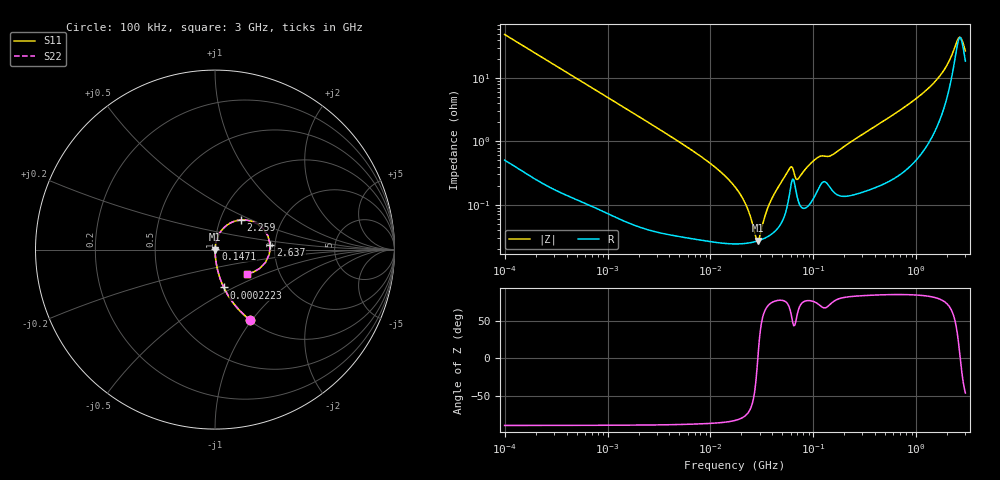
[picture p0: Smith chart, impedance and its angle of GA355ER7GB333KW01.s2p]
!Murata Part Number: GA355ER7GB333KW01
!These Parameters are Measured in Series Mode Connection
!Data Generated on Jun 19, 2026
!  o--ll--o
!Port1  Port2
!  o------o
!Operation Temp=25[degC], DC Bias Voltage=0[V]
!Freq. Start=100[kHz] Stop=3[GHz] 401[Steps]
# Hz S RI R 50
!Freq.(Hz) S11(Real) S11(Imag) S21(Real) S21(Imag) S12(Real) S12(Imag) S22(Real) S22(Imag)
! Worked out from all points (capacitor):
!   401 points, 100 kHz to 3 GHz, reference 50 ohm
!   read as one part in series: C = 32.4 nF near 105.3 kHz
!   lowest |Z| = 26.9 mohm at 29 MHz (marker M1)
!   series resonance near 28.86 MHz, so ESL is about 940 pH
!   S11 on the Smith chart (normalised r, x): 100 kHz: 1.01, -0.98; 222.3 kHz: 1.00, -0.44; 147.1 MHz: 1.00, +0.01; 2.259 GHz: 1.25, +0.43; 2.637 GHz: 1.88, +0.11; 3 GHz: 1.37, -0.39
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100000  0.1965 -0.3923  0.8035 0.3923  0.8035 0.3923  0.1965 -0.3923
222319  0.0489 -0.2105  0.9511 0.2105  0.9511 0.2105  0.0489 -0.2105
562235  0.00879 -0.0873  0.9912 0.0873  0.9912 0.0873  0.00879 -0.0873
3161081  0.000607 -0.0157  0.9994 0.0157  0.9994 0.0157  0.000607 -0.0157
1.008119e7  0.000279 -0.00442  0.9997 0.00442  0.9997 0.00442  0.000279 -0.00442
1.77727e7  0.000243 -0.00179  0.9998 0.00179  0.9998 0.00179  0.000243 -0.00179
2.241242e7  0.000246 -0.000916  0.9998 0.000916  0.9998 0.000916  0.000246 -0.000916
2.754426e7  0.000262 -0.000168  0.9997 0.000168  0.9997 0.000168  0.000262 -0.000168
2.900125e7  0.000268 1.85e-05  0.9997 -1.85e-05  0.9997 -1.85e-05  0.000268 1.85e-05
3.850681e7  0.000336 0.00109  0.9997 -0.00109  0.9997 -0.00109  0.000336 0.00109
5.815973e7  0.00136 0.00337  0.9986 -0.00337  0.9986 -0.00337  0.00136 0.00337
6.123616e7  0.00222 0.0033  0.9978 -0.0033  0.9978 -0.0033  0.00222 0.0033
7.147675e7  0.00114 0.00231  0.9989 -0.00231  0.9989 -0.00231  0.00114 0.00231
9.738194e7  0.00117 0.00457  0.9988 -0.00457  0.9988 -0.00457  0.00117 0.00457
1.166348e8  0.00204 0.00545  0.998 -0.00545  0.998 -0.00545  0.00204 0.00545
1.470833e8  0.00185 0.00563  0.9982 -0.00563  0.9982 -0.00563  0.00185 0.00563
5.475153e8  0.00291 0.0238  0.9971 -0.0238  0.9971 -0.0238  0.00291 0.0238
1.384641e9  0.0161 0.0726  0.9839 -0.0726  0.9839 -0.0726  0.0161 0.0726
1.886474e9  0.0511 0.1232  0.9489 -0.1232  0.9489 -0.1232  0.0511 0.1232
2.259438e9  0.1439 0.1653  0.8561 -0.1653  0.8561 -0.1653  0.1439 0.1653
2.637286e9  0.3077 0.0271  0.6923 -0.0271  0.6923 -0.0271  0.3077 0.0271
3e9  0.1791 -0.1346  0.8209 0.1346  0.8209 0.1346  0.1791 -0.1346
